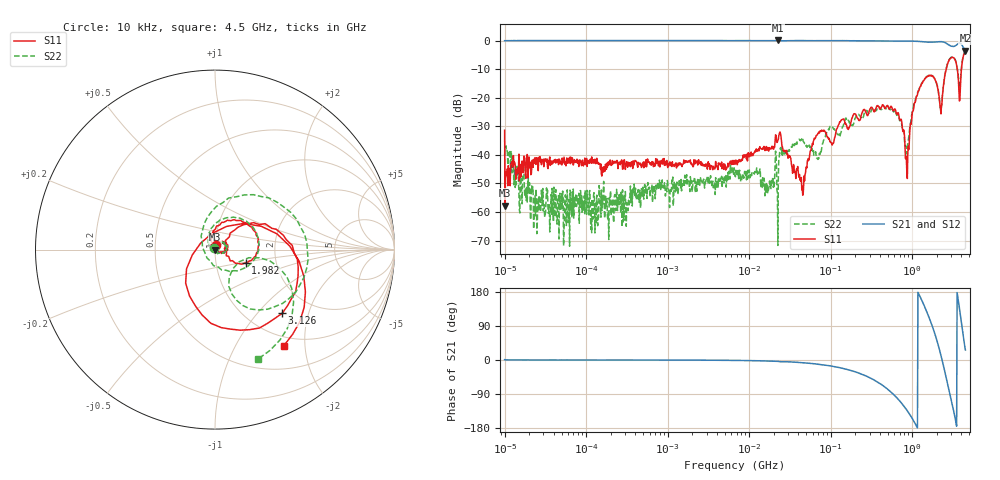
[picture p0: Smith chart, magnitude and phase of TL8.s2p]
!Siglent Technologies,SNA5004A,SNA5XCED5R0097,V1.0.0.2.10.R9
!Date: 2024-11-24 17:04:47
!Data & Calibration Information:
!Freq	S11:F2(ON)	S21:F2(ON)	S12:F2(ON)	S22:F2(ON)
# Hz S DB R 50
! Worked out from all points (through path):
!   1001 points, 10 kHz to 4.5 GHz, reference 50 ohm
!   highest |S21| = 0.10 dB at 22.8 MHz (marker M1); lowest = -3.5 dB at 4.5 GHz (marker M2)
!   group delay of S21, straight-line fit = 428 ps
!   lowest |S11| = -57.7 dB at 10.13 kHz (marker M3), VSWR 1.00, Z = 49.9 - j0.0361 ohm
!   |S11| at or under -10 dB: start of sweep to 2.607 GHz; 3.579 GHz to 4.025 GHz (446 MHz wide, 11.7 % of centre)
!   |S22| runs from -72.0 to -3.7 dB; largest |S21 - S12| = 0.024
!   S11 on the Smith chart (normalised r, x): 10 kHz: 1.01, +0.05; 1.982 GHz: 1.39, -0.21; 3.126 GHz: 1.42, -1.37; 4.5 GHz: 0.85, -1.61
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10000  -31.36 79.8  0.01 0.8  -0.02 0.9  -40.25 126.3
10131.02  -57.73 -163.8  -0.01 0.3  -0.06 0.2  -37.65 120.3
10812.33  -44.84 -45.8  0.04 0.1  -0.02 0.3  -39.01 88.8
24233.63  -43.33 11.3  0.05 0.1  -0.00 0.1  -51.94 108.8
87919.76  -43.77 11.4  0.06 0.0  -0.00 -0.1  -53.78 -67.2
772988.4  -43.84 17.2  0.05 -0.1  -0.00 -0.2  -52.27 -59.9
6708204  -43.28 64.0  0.04 -1.1  -0.03 -1.2  -47.32 -134.4
2.280385e7  -34.60 123.4  0.10 -3.8  0.02 -3.8  -48.32 118.2
4.487199e7  -51.01 123.6  0.05 -7.2  -0.06 -7.1  -34.59 86.1
5.897837e7  -37.07 49.8  0.01 -9.4  -0.06 -9.4  -37.75 110.2
2.313556e8  -27.67 50.0  -0.03 -36.0  -0.12 -35.8  -26.53 59.1
5.185364e8  -23.82 12.0  -0.10 -79.9  -0.16 -79.6  -23.60 8.4
8.727859e8  -48.27 96.7  -0.12 -134.2  -0.17 -133.9  -37.81 -163.2
1.192847e9  -17.53 85.6  -0.23 176.1  -0.28 176.4  -17.60 94.1
1.609195e9  -12.13 22.4  -0.51 112.8  -0.56 113.1  -12.15 25.3
1.981801e9  -14.63 -23.5  -0.42 56.4  -0.48 56.9  -14.80 -37.7
2.409119e9  -16.24 44.8  -0.42 -12.9  -0.49 -12.3  -16.14 112.8
2.74404e9  -7.94 8.0  -1.25 -66.3  -1.29 -65.6  -7.63 44.0
3.125522e9  -5.75 -43.5  -2.00 -120.1  -2.05 -119.3  -5.66 -11.5
3.653937e9  -12.09 -131.1  -1.05 162.5  -1.11 163.4  -11.53 -69.1
4.002521e9  -10.78 26.7  -1.17 99.9  -1.22 101.3  -10.16 -11.5
4.5e9  -3.62 -54.4  -3.53 26.3  -3.56 27.7  -3.67 -68.6
